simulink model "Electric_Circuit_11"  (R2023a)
settings: Solver=VariableStepAuto  StartTime=0.0  StopTime=10.0  RelTol=1e-3
libraries: fl_lib x12

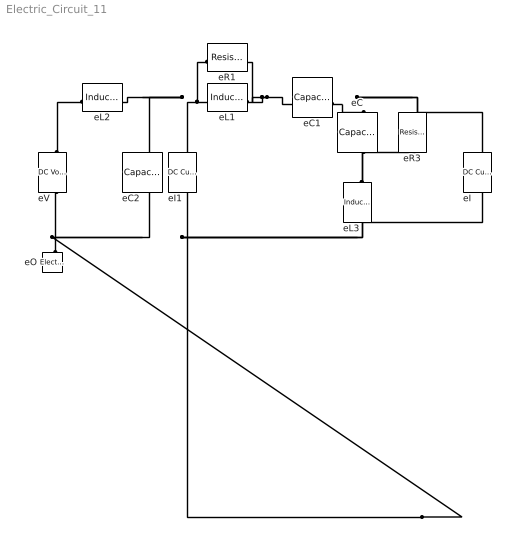
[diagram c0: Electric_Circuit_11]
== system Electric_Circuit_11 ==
  eC : fl_lib/Electrical/Electrical Elements/Capacitor  c=1e-6 F  r=1e-6 Ohm  g=0 1/Ohm  i_specify=off  i_priority=None  i=0 A  i_nominal_specify=off  i_nominal_unit=A  i_nominal_value=1  v_specify=off  v_priority=None  v=0 V  v_nominal_specify=off  v_nominal_unit=V  v_nominal_value=1  vc_specify=off  vc_priority=High  vc=0 V  vc_nominal_specify=off  vc_nominal_unit=V  vc_nominal_value=1
  eC1 : fl_lib/Electrical/Electrical Elements/Capacitor  c=1e-6 F  r=1e-6 Ohm  g=0 1/Ohm  i_specify=off  i_priority=None  i=0 A  i_nominal_specify=off  i_nominal_unit=A  i_nominal_value=1  v_specify=off  v_priority=None  v=0 V  v_nominal_specify=off  v_nominal_unit=V  v_nominal_value=1  vc_specify=off  vc_priority=High  vc=0 V  vc_nominal_specify=off  vc_nominal_unit=V  vc_nominal_value=1
  eC2 : fl_lib/Electrical/Electrical Elements/Capacitor  c=1e-6 F  r=1e-6 Ohm  g=0 1/Ohm  i_specify=off  i_priority=None  i=0 A  i_nominal_specify=off  i_nominal_unit=A  i_nominal_value=1  v_specify=off  v_priority=None  v=0 V  v_nominal_specify=off  v_nominal_unit=V  v_nominal_value=1  vc_specify=off  vc_priority=High  vc=0 V  vc_nominal_specify=off  vc_nominal_unit=V  vc_nominal_value=1
  eI : fl_lib/Electrical/Electrical Sources/DC Current Source  i0=1 A
  eI1 : fl_lib/Electrical/Electrical Sources/DC Current Source  i0=1 A
  eL1 : fl_lib/Electrical/Electrical Elements/Inductor  l=1e-6 H  r=0 Ohm  g=1e-9 1/Ohm  i_specify=off  i_priority=None  i=0 A  i_nominal_specify=off  i_nominal_unit=A  i_nominal_value=1  v_specify=off  v_priority=None  v=0 V  v_nominal_specify=off  v_nominal_unit=V  v_nominal_value=1  i_L_specify=off  i_L_priority=High  i_L=0 A  i_L_nominal_specify=off  i_L_nominal_unit=A  i_L_nominal_value=1
  eL2 : fl_lib/Electrical/Electrical Elements/Inductor  l=1e-6 H  r=0 Ohm  g=1e-9 1/Ohm  i_specify=off  i_priority=None  i=0 A  i_nominal_specify=off  i_nominal_unit=A  i_nominal_value=1  v_specify=off  v_priority=None  v=0 V  v_nominal_specify=off  v_nominal_unit=V  v_nominal_value=1  i_L_specify=off  i_L_priority=High  i_L=0 A  i_L_nominal_specify=off  i_L_nominal_unit=A  i_L_nominal_value=1
  eL3 : fl_lib/Electrical/Electrical Elements/Inductor  l=1e-6 H  r=0 Ohm  g=1e-9 1/Ohm  i_specify=off  i_priority=None  i=0 A  i_nominal_specify=off  i_nominal_unit=A  i_nominal_value=1  v_specify=off  v_priority=None  v=0 V  v_nominal_specify=off  v_nominal_unit=V  v_nominal_value=1  i_L_specify=off  i_L_priority=High  i_L=0 A  i_L_nominal_specify=off  i_L_nominal_unit=A  i_L_nominal_value=1
  eO : fl_lib/Electrical/Electrical Elements/Electrical Reference
  eR1 : fl_lib/Electrical/Electrical Elements/Resistor  R=1 Ohm  i_specify=off  i_priority=None  i=0 A  i_nominal_specify=off  i_nominal_unit=A  i_nominal_value=1  v_specify=off  v_priority=None  v=0 V  v_nominal_specify=off  v_nominal_unit=V  v_nominal_value=1
  eR3 : fl_lib/Electrical/Electrical Elements/Resistor  R=1 Ohm  i_specify=off  i_priority=None  i=0 A  i_nominal_specify=off  i_nominal_unit=A  i_nominal_value=1  v_specify=off  v_priority=None  v=0 V  v_nominal_specify=off  v_nominal_unit=V  v_nominal_value=1
  eV : fl_lib/Electrical/Electrical Sources/DC Voltage Source  v0=1 V
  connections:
  eO/LConn1 -- eC2/RConn1 -- eI/RConn1 -- eL3/RConn1 -- eI1/RConn1 -- eV/RConn1
  eR1/LConn1 -- eI1/LConn1 -- eC2/LConn1 -- eL2/RConn1 -- eL1/LConn1
  eL1/RConn1 -- eR1/RConn1 -- eC1/LConn1
  eC1/RConn1 -- eI/LConn1 -- eR3/LConn1 -- eC/LConn1
  eV/LConn1 -- eL2/LConn1
  eL3/LConn1 -- eC/RConn1 -- eR3/RConn1
